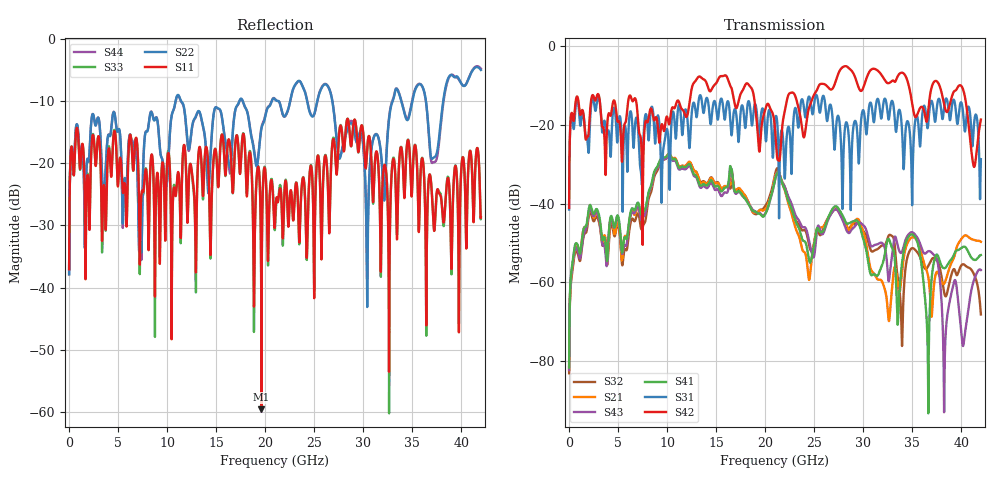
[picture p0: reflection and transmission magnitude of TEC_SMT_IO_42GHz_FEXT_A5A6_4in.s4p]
!! CHANNEL DESCRIPTION: Next Generation 28Gbps High Density SMT I/O Connector
!!  with 4" 5-6-5 Megatron 6 Stripline trace on host side and 1.25" 7-5-7 Megtron 6 Microstrip trace on plug side at 14GHz
!! HOST PCB DESCRIPTION: PCB thickness 2.86 mm, Nelco 4000-13SI (Dk 3.32, Df 0.010)
!!  23 Layer Board, 12 GND planes, 2 Layer route-out on Layers 10,12, 8 mil stub on vias
!!  Pairs on following layers
!!  Layer 12 - A5A6
!! CONNECTOR DESCRIPTION:  Next Generation 28Gbps High Density SMT I/O Connector
!! PLUG-IN CARD DESCRIPTION:  PCB thickness 1mm thick, Nelco 4000-13SI (Dk 3.32, Df 0.010)
!!  6 Layer Board, 4 GND planes, 0.35 x 1.4mm mating pads
!!  Micro-strip diff traces referenced to GND plane 3mils down, 2nd GND plane 15mils from top of board
!!  PCB GND planes are symmetric
!! MODEL DESCRIPTION: TE Connectivity S-parameter model produced from Macro-model
!! MODEL DATE: 9/25/2014 CR1a_GC1i, VR6&12_4
!! MODEL STATUS: Developmental
!! MODEL GEOMETRY: 2 Rows - Rows A, B. 3 pairs in each row, 6 total pairs
!! MODEL FREQUENCY RANGE: DC to 42 GHz in 10 MHz frequency steps
!! MODEL EDGE RATE LIMITATION: 11.90 ps (Using conservative 0.5/Fmax rule of thumb)
!! TIME-DOMAIN TRANSFORM CAUTIONS:
!! 1.) Do not simulate transient edge rates faster than the number listed above.  Edge
!!  rates faster than this number contain significant spectral content at frequencies
!!  above the model's highest frequency.
!! 2.) Even when simulating edge rates that are slower than the number listed above, be
!!  aware that the best time resolution possible with a direct iFFT is (1 / 2Fmax).
!!  As a result, time resolution is typically not adequate for most time-domain
!!  simulations unless tricks such as frequency-domain zero-padding and windowing are
!!  used to minimize leakage and aliasing.
!! 3.) Because the model has a uniform frequency step, a direct iFFT will result in an
!!  impulse that that has a time length given by either (1 / Fstep) or (1 / 2Fstep),
!!  depending on the transform being used.  Care has been taken in selecting the
!!  frequency step to ensure a settled impulse response for the model.  Therefore,
!!  convolution with the model's impulse response should present no issues.  However,
!!  if directly concatenating s-parameter models in the frequency domain a user must
!!  either interpolate necessary interim frequencies or complete impulse response
!!  zero-padding.  Impulse response zero-padding is more difficult, but more accurate.
!! PORT DEFINITIONS:
!! Port  1  ----->  Host, Bot Row  A5  B5  Module, Top Row  <-----  Port  2
!! Port  3  ----->  Host, Bot Row  A6  B6  Module, Top Row  <-----  Port  4
# Hz S MA R 50
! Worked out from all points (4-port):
!   4200 points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, 10 MHz to 42 GHz, reference 50 ohm
!   strongest paths, dB at 10 MHz, 10.51 GHz, 21.01 GHz, 31.51 GHz, 42 GHz:
!     S42: -41.1, -15.7, -21.2, -6.3, -18.7
!     S31: -41.5, -17.7, -18.8, -13.5, -28.8
!     S41: -81.6, -28.6, -33.9, -58.1, -53.1
!     S43: -82.3, -29.1, -33.9, -50.3, -56.9
!     S21: -82.2, -28.4, -33.2, -59.3, -49.7
!     S32: -83.0, -28.6, -32.6, -51.5, -68.1
!   lowest |S11| = -59.5 dB at 19.62 GHz (marker M1), VSWR 1.00, Z = 49.9 + j0.0506 ohm
!   |S11| at or under -10 dB: start of sweep to end of sweep
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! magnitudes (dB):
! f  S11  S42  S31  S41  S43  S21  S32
! 10 MHz  -37.1  -41.1  -41.5  -81.6  -82.3  -82.2  -83.0
! 9.5 GHz  -20.1  -19.9  -31.4  -28.4  -28.8  -28.6  -29.1
! 19.62 GHz  -59.5  -20.8  -16.7  -43.0  -42.8  -41.7  -41.5
! 35.09 GHz  -20.0  -16.1  -27.5  -48.0  -47.4  -48.5  -51.3
! 36.59 GHz  -25.3  -17.5  -20.7  -78.9  -52.2  -58.1  -56.0
! 38.3 GHz  -28.3  -15.3  -14.7  -56.4  -81.5  -60.1  -63.0
! 42 GHz  -28.7  -18.7  -28.8  -53.1  -56.9  -49.7  -68.1
